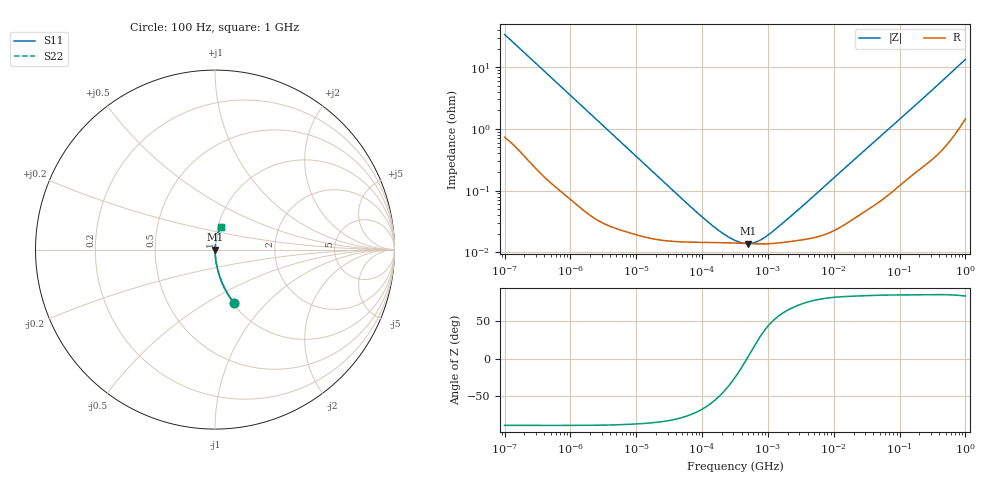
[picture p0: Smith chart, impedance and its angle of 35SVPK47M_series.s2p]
!  *** S-Parameter ***
!  Copyright (C) Panasonic Industry
!  Conductive Polymer Aluminum Soild Capacitor (OS-CON)
!  Parts No. 35SVPK47M
!  Connection Mode : Series
!  1  o---||---o  2
!  GND o--------o GND
!  Conditions : Temperature = 20 degC  DC Bias = 0 V
! Frequency Range : 100Hz  -  1GHz  [ 401 Steps ]
# Hz S RI R 50
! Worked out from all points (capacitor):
!   401 points, 100 Hz to 1 GHz, reference 50 ohm
!   read as one part in series: C = 46.9 uF near 108.4 Hz
!   lowest |Z| = 13.8 mohm at 492.6 kHz (marker M1)
!   series resonance near 479 kHz, so ESL is about 2.4 nH
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100  0.1075 -0.2991  0.8925 0.2991  0.8925 0.2991  0.1075 -0.2991
108.3927  0.0938 -0.2808  0.9062 0.2808  0.9062 0.2808  0.0938 -0.2808
168.8496  0.043 -0.1924  0.957 0.1924  0.957 0.1924  0.043 -0.1924
321.7363  0.0133 -0.1052  0.9867 0.1052  0.9867 0.1052  0.0133 -0.1052
638.2635  0.00399 -0.054  0.996 0.054  0.996 0.054  0.00399 -0.054
1487.647  0.00105 -0.0235  0.9989 0.0235  0.9989 0.0235  0.00105 -0.0235
22130.95  0.000161 -0.00161  0.9998 0.00161  0.9998 0.00161  0.000161 -0.00161
68391.16  0.000146 -0.000515  0.9999 0.000515  0.9999 0.000515  0.000146 -0.000515
130316.7  0.000144 -0.000256  0.9999 0.000256  0.9999 0.000256  0.000144 -0.000256
211348.9  0.000143 -0.000138  0.9999 0.000138  0.9999 0.000138  0.000143 -0.000138
316227.8  0.000141 -6.56e-05  0.9999 6.56e-05  0.9999 6.56e-05  0.000141 -6.56e-05
402717  0.00014 -2.71e-05  0.9999 2.71e-05  0.9999 2.71e-05  0.00014 -2.71e-05
492606.3  0.000138 4.41e-06  0.9999 -4.41e-06  0.9999 -4.41e-06  0.000138 4.41e-06
679986  0.000137 5.72e-05  0.9999 -5.72e-05  0.9999 -5.72e-05  0.000137 5.72e-05
977237.2  0.000137 0.000126  0.9999 -0.000126  0.9999 -0.000126  0.000137 0.000126
1788546  0.000145 0.000279  0.9999 -0.000279  0.9999 -0.000279  0.000145 0.000279
4704354  0.00017 0.000755  0.9998 -0.000755  0.9998 -0.000755  0.00017 0.000755
6.99842e7  0.000974 0.0101  0.999 -0.0101  0.999 -0.0101  0.000974 0.0101
3.368992e8  0.00544 0.0451  0.9946 -0.0451  0.9946 -0.0451  0.00544 0.0451
5.688529e8  0.0118 0.0747  0.9882 -0.0747  0.9882 -0.0747  0.0118 0.0747
9.225714e8  0.0267 0.1176  0.9733 -0.1176  0.9733 -0.1176  0.0267 0.1176
1e9  0.0307 0.1265  0.9693 -0.1265  0.9693 -0.1265  0.0307 0.1265
